FUNCTION_BLOCK Example18_jogging //4x3 flyways 1 xbot - jogging, jogging short axis
VAR_INPUT
	Execute : BOOL;
END_VAR
VAR_OUTPUT
	Done : BOOL;
END_VAR
VAR_IN_OUT
	PM_Controller : PMControllerType;	// the planar motor controller to use
END_VAR
VAR
	PMC_XYMotion1 : PMC_XYMotion;
	PMC_JogVelocity1 : PMC_JogVelocity;
	Delay1 : Delay; 
	PMC_JogVelocity2 : PMC_JogVelocity;
	Delay2 : Delay;
	PMC_JogVelocity3 : PMC_JogVelocity;
	Delay3 : Delay;
	PMC_JogVelocity4 : PMC_JogVelocity;
	
	Delay4 : Delay;
	PMC_JogShortAxis1 : PMC_JogShortAxis;
	Delay5 : Delay;
	PMC_JogshortAxis2 : PMC_JogShortAxis;
	Delay6 : Delay;
	PMC_JogShortAxis3 : PMC_JogShortAxis;
	Delay7 : Delay;
	PMC_JogshortAxis4 : PMC_JogShortAxis;
END_VAR

//4x3 flyways 1 xbot - jogging, jogging short axis

//move xbot 1 to 120,120
PMC_XYMotion1(Execute := Execute,cmdLB := 1,XbotID := 1,Mode := 0,Type_ := 0,PosX := 0.12,PosY := 0.12,EndVel := 0,MaxVel := 1,MaxAcc := 10,PM_Controller := PM_Controller);

//jog xbot 1 up and right
PMC_JogVelocity1(Execute := PMC_XYMotion1.Done,XbotID := 1,Enable := TRUE,Direction := 0.7854,Velocity := 0.05,PM_Controller := PM_Controller);
Delay1(Execute := PMC_JogVelocity1.Done,Cycles := 10000);

//stop xbot 1 jogging
PMC_JogVelocity2(Execute := Delay1.Done,XbotID := 1,Enable := FALSE,Direction := 3.927,Velocity := 0.05,PM_Controller := PM_Controller);
Delay2(Execute := PMC_JogVelocity2.Done,Cycles := 500);

//jog xbot 1 down and left
PMC_JogVelocity3(Execute := Delay2.Done,XbotID := 1,Enable := TRUE,Direction := 3.927,Velocity := 0.05,PM_Controller := PM_Controller);
Delay3(Execute := PMC_JogVelocity3.Done,Cycles := 10000);

//stop xbot 1 jogging
PMC_JogVelocity4(Execute := Delay3.Done,XbotID := 1,Enable := FALSE,Direction := 3.927,Velocity := 0.05,PM_Controller := PM_Controller);
Delay4(Execute := PMC_JogVelocity4.Done,Cycles := 500);

//jog xbot 1 counterclockwise (positive Rz)
PMC_JogShortAxis1(Execute := Delay4.Done,XbotID := 1,Enable := TRUE,AxisID := 3,Velocity := 0.001,PM_Controller := PM_Controller);
Delay5(Execute := PMC_JogShortAxis1.Done,Cycles := 7500);

//stop xbot 1 jogging
PMC_JogShortAxis2(Execute := Delay5.Done,XbotID := 1,Enable := FALSE,AxisID := 3,Velocity := 0.001,PM_Controller := PM_Controller);
Delay6(Execute := PMC_JogShortAxis2.Done,Cycles := 500);

//jog xbot 1 clockwise (negative Rz)
PMC_JogShortAxis3(Execute := Delay6.Done,XbotID := 1,Enable := TRUE,AxisID := 3,Velocity := -0.001,PM_Controller := PM_Controller);
Delay7(Execute := PMC_JogShortAxis3.Done,Cycles := 7500);

//stop xbot 1 jogging
PMC_JogshortAxis4(Execute := Delay7.Done,XbotID := 1,Enable := FALSE,AxisID := 3,Velocity := -0.001,PM_Controller := PM_Controller);

Done := PMC_JogshortAxis4.Done;

END_FUNCTION_BLOCK
